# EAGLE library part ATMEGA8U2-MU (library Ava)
Pakage: TQFP32
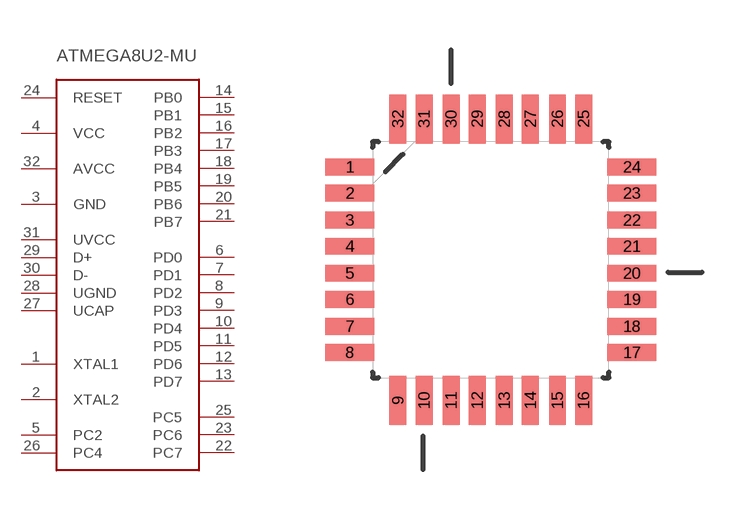
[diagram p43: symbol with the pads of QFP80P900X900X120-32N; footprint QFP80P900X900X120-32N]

Designator prefix -

## ATMEGA8U2-MU  [QFP80P900X900X120-32N]
1  XTAL1
2  XTAL2
3  GND
4  VCC
5  PC2
6  PD0
7  PD1
8  PD2
9  PD3
10  PD4
11  PD5
12  PD6
13  PD7
14  PB0
15  PB1
16  PB2
17  PB3
18  PB4
19  PB5
20  PB6
21  PB7
22  PC7
23  PC6
24  RESET
25  PC5
26  PC4
27  UCAP
28  UGND
29  D+
30  D-
31  UVCC
32  AVCC

## Footprint QFP80P900X900X120-32N (pad centres in mm)
smd 1.473 x 0.508: 1 -4.242,2.794; 2 -4.242,2.007; 3 -4.242,1.194; 4 -4.242,0.406; 5 -4.242,-0.406; 6 -4.242,-1.194; 7 -4.242,-2.007; 8 -4.242,-2.794; 17 4.242,-2.794; 18 4.242,-2.007; 19 4.242,-1.194; 20 4.242,-0.406; 21 4.242,0.406; 22 4.242,1.194; 23 4.242,2.007; 24 4.242,2.794
smd 0.508 x 1.473: 9 -2.794,-4.242; 10 -2.007,-4.242; 11 -1.194,-4.242; 12 -0.406,-4.242; 13 0.406,-4.242; 14 1.194,-4.242; 15 2.007,-4.242; 16 2.794,-4.242; 25 2.794,4.242; 26 2.007,4.242; 27 1.194,4.242; 28 0.406,4.242; 29 -0.406,4.242; 30 -1.194,4.242; 31 -2.007,4.242; 32 -2.794,4.242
